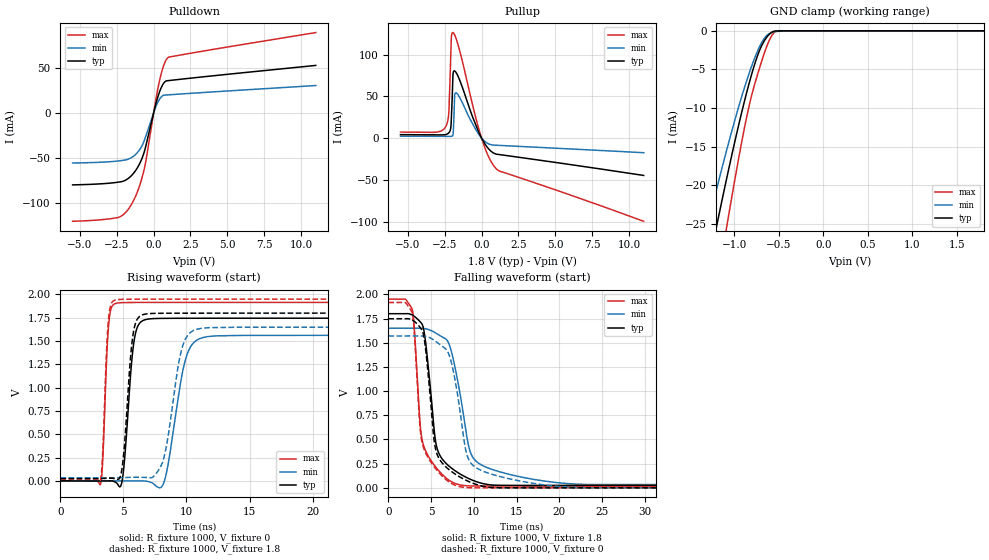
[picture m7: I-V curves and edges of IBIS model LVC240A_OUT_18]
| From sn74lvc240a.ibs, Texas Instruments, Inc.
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[Model]   LVC240A_OUT_18
Model_type  3-state
Enable   Active-Low
Vref =   0
Rref =   1000
Cref =   30p
Vmeas =   0.9
| variable   typ   min   max
C_comp   5.37pF   5.23pF   5.85pF
| C_pullup   6.94pF   5.96pF   7.46pF
| C_pulldown   6.77pF   5.28pF   7.89pF
| C_tri-state   5.37pF   5.23pF   5.85pF
[Temperature Range]   40   100   -40
| Ambient temperature   25   85   -40
[Voltage range]   1.8   1.65   1.95
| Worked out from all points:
|   slope of the pulldown table from 0 to 0.27 V, typ, clamps not added: 16.1 ohm
|   slope of the pullup table from 0 to 0.27 V, typ, clamps not added: 33.2 ohm
|   GND clamp passes 1 mA (typ) near -0.65 V on its own axis
|   rising waveform, R_fixture 1000, V_fixture 0: 20-80 % time 582ps typ, 1.12ns min, 341ps max; typ from 0 V to 1.75 V
|   falling waveform, R_fixture 1000, V_fixture 1.8: 20-80 % time 1.37ns typ, 2.05ns min, 1.15ns max; typ from 1.8 V to 0.026 V
|   rising waveform, R_fixture 1000, V_fixture 1.8: 20-80 % time 570ps typ, 1.09ns min, 335ps max; typ from 0.025 V to 1.8 V
|   falling waveform, R_fixture 1000, V_fixture 0: 20-80 % time 1.29ns typ, 1.82ns min, 1.16ns max; typ from 1.75 V to 0 V
[GND Clamp]
| LVC240A_OUT_18
|   Voltage   I(typ)   I(min)   I(max)
-5.5V     -311.6mA   -259.3mA   -396.4mA
-1.3V     -31.17mA   -25.35mA   -40.84mA
-1.215V   -26.32mA   -21.36mA   -34.65mA
-1.175V   -24.09mA   -19.52mA   -31.79mA
-1.1V     -19.99mA   -16.16mA   -26.53mA
-1.06V    -17.86mA   -14.42mA   -23.79mA
-880mV    -8.928mA   -7.206mA   -12.33mA
-765mV    -4.161mA   -3.399mA   -6.744mA
-655mV    -1.171mA   -880.6uA   -2.683mA
-590mV    -295.4uA   -275.9uA   -882.9uA
-540mV    -28.91uA   -111.9uA   -128.1uA
1.8V      35.25pA    10.02nA    -1.385nA
[Pulldown]
| LVC240A_OUT_18
|   Voltage   I(typ)   I(min)   I(max)
-5.5V     -79.86mA   -55.62mA   -120.2mA
-2.405V   -76.84mA   -53.37mA   -115.9mA
-1.95V    -74.97mA   -52.33mA   -111.2mA
-1.505V   -69.56mA   -49.58mA   -101.4mA
-1.04V    -59.1mA    -42.78mA   -84.85mA
-665mV    -44.74mA   -31.97mA   -64.09mA
-520mV    -36.04mA   -25.31mA   -52.64mA
70mV      4.78mA     3.284mA    7.076mA
355mV     21.12mA    13.82mA    32.13mA
675mV     32.63mA    19.38mA    52.09mA
970mV     35.59mA    19.83mA    61.12mA
11V       52.47mA    30.19mA    88.86mA
[Pullup]
| LVC240A_OUT_18
|   Voltage   I(typ)   I(min)   I(max)
-5.5V     4.132mA    2.28mA     7.221mA
-2.42V    4.318mA    2.093mA    14.19mA
-2.225V   6.276mA    2.078mA    30.14mA
-2.085V   12.97mA    2.077mA    101.8mA
-2.045V   25.72mA    2.109mA    121.9mA
-1.945V   74.01mA    3.627mA    126.3mA
-1.895V   79.92mA    16.59mA    125.6mA
-1.83V    80.38mA    50.38mA    123.6mA
-1.73V    78.5mA     54.05mA    119.2mA
-25mV     874.8uA    531.1uA    1.42mA
995mV     -19.19mA   -8.546mA   -36.64mA
11V       -44.72mA   -17.52mA   -99.61mA
[Ramp]
| LVC240A_OUT_18
| variable   typ   min   max
dV/dt_r   1.08/6.03E-10   0.98/1.16E-09   1.17/3.53E-10
dV/dt_f   1.07/1.37E-09   0.97/2.04E-09   1.16/1.16E-09
R_load = 1000
[Rising Waveform]
| LVC240A_OUT_18
R_fixture =   1000
C_fixture =   0
L_fixture =   0
V_fixture =   0
V_fixture_min = 0
V_fixture_max = 0
|   Time   V(typ)   V(min)   V(max)
0s        658.2pV    3.523nV    28.78nV
3.18ns    -248.8uV   -82.74uV   -33.67mV
3.82ns    192.6uV    -188.4uV   1.667V
4.405ns   -17.13mV   -156.4uV   1.905V
5.89ns    1.541V     248.1uV    1.914V
6.725ns   1.73V      -1.208mV   1.914V
8.175ns   1.744V     -29.14mV   1.915V
9.895ns   1.745V     1.29V      1.915V
11.3ns    1.745V     1.538V     1.915V
50ns      1.746V     1.563V     1.915V
[Falling Waveform]
| LVC240A_OUT_18
R_fixture =   1000
C_fixture =   0
L_fixture =   0
V_fixture =   1.8
V_fixture_min = 1.65
V_fixture_max = 1.95
|   Time   V(typ)   V(min)   V(max)
0s        1.8V       1.65V      1.95V
2.82ns    1.785V     1.651V     1.835V
3.695ns   1.718V     1.649V     682.4mV
3.975ns   1.686V     1.649V     483.7mV
5.61ns    439.1mV    1.596V     206.9mV
6.925ns   237.9mV    1.517V     89.93mV
7.685ns   184mV      1.291V     49.94mV
9.595ns   88.11mV    366.9mV    19.75mV
12.18ns   28.68mV    188.5mV    19.07mV
50ns      25.51mV    33.86mV    18.78mV
[Rising Waveform]
| LVC240A_OUT_18
R_fixture =   1000
C_fixture =   0
L_fixture =   0
V_fixture =   1.8
V_fixture_min = 1.65
V_fixture_max = 1.95
|   Time   V(typ)   V(min)   V(max)
0s        25.49mV    33.75mV    18.77mV
3.16ns    25.86mV    33.63mV    440.2uV
3.79ns    28.83mV    33.88mV    1.7V
4.335ns   20.83mV    34.37mV    1.939V
4.925ns   173.4mV    35.11mV    1.948V
5.795ns   1.599V     38.61mV    1.949V
6.585ns   1.785V     38.12mV    1.949V
8.08ns    1.798V     194mV      1.95V
10.84ns   1.799V     1.628V     1.95V
50ns      1.8V       1.65V      1.95V
[Falling Waveform]
| LVC240A_OUT_18
R_fixture =   1000
C_fixture =   0
L_fixture =   0
V_fixture =   0
V_fixture_min = 0
V_fixture_max = 0
|   Time   V(typ)   V(min)   V(max)
0s        1.748V     1.57V      1.916V
2.82ns    1.733V     1.57V      1.796V
3.665ns   1.663V     1.569V     668.9mV
3.955ns   1.627V     1.569V     464.3mV
5.515ns   402.8mV    1.516V     199.5mV
6.935ns   200.1mV    1.409V     71.73mV
7.71ns    148.3mV    1.155V     31.05mV
9.29ns    69.75mV    314.4mV    2.15mV
12.02ns   3.567mV    142.7mV    290.3uV
50ns      27.4uV     105.1uV    9.794uV
